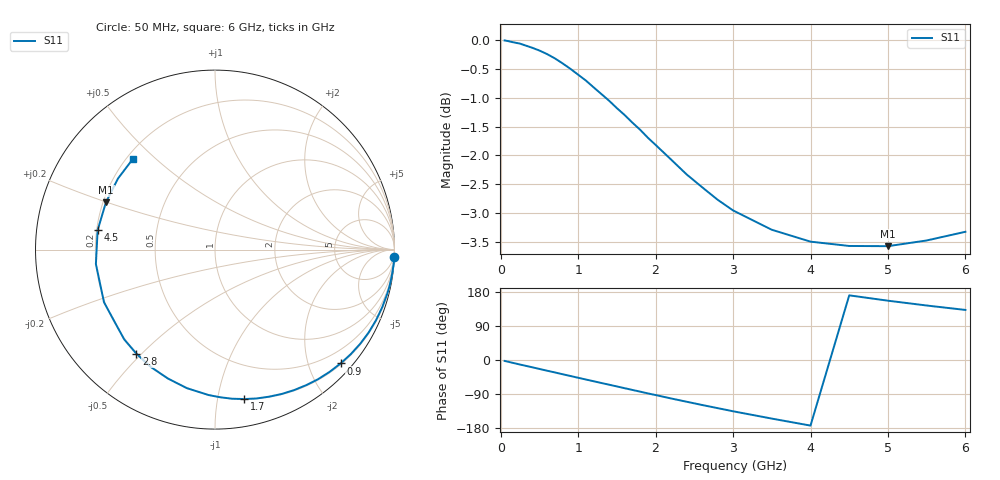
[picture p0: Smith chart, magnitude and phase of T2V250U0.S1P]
! SIEMENS Discrete & RF Semiconductors
! BAS70-04W
! Si Schottky Diode in SOT323
! VR = 0.25 V
! S-Parameters:  November  1997
# GHz  S  MA  R  50
!  f  S11
! GHz  MAG  ANG
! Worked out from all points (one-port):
!   34 points, 50 MHz to 6 GHz, reference 50 ohm
!   lowest |S11| = -3.6 dB at 5 GHz (marker M1), VSWR 4.92, Z = 10.6 + j9.95 ohm
!   |S11| at or under -10 dB: nowhere
!   S11 on the Smith chart (normalised r, x): 50 MHz: 0, -48; 900 MHz: 0.22, -2.58; 1.7 GHz: 0.20, -1.19; 2.8 GHz: 0.20, -0.48; 4.5 GHz: 0.20, +0.08; 6 GHz: 0.22, +0.43
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0.05  0.9998 -2.4
0.25  0.9934 -12.0
0.4  0.9856 -18.9
0.5  0.9798 -23.6
0.6  0.9727 -28.3
0.7  0.9644 -32.9
0.8  0.9548 -37.6
0.9  0.9446 -42.2
1  0.9335 -46.9
1.1  0.9226 -51.5
1.2  0.9101 -56.1
1.3  0.8981 -60.7
1.4  0.8861 -65.2
1.6  0.8611 -74.4
1.7  0.8482 -79.0
1.8  0.8362 -83.5
2  0.8112 -92.5
2.2  0.7877 -101.5
2.4  0.7647 -110.1
2.6  0.7454 -118.7
2.8  0.727 -127.0
3  0.7115 -135.3
3.5  0.6845 -154.6
4  0.6684 -173.1
4.5  0.6627 170.6
5  0.6624 156.5
5.5  0.67 143.8
6  0.6817 132.1
